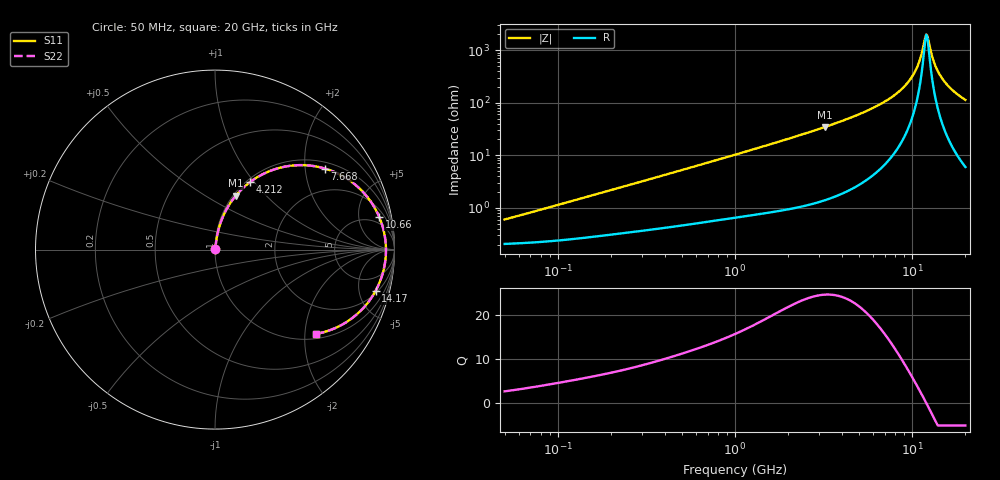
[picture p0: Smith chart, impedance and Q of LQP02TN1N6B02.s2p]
!Murata Part Number: LQP02TN1N6B02
!These Parameters are Measured in Series Mode Connection
!  o--[Z]--o
!Port1  Port2
!  o-------o
!Freq. Start=50[MHz] Stop=20[GHz], 401[Steps]
# Hz S RI R 50
!Freq.(Hz) S11(Real) S11(Imag) S21(Real) S21(Imag) S12(Real) S12(Imag) S22(Real) S22(Imag)
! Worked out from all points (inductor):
!   401 points, 50 MHz to 20 GHz, reference 50 ohm
!   read as one part in series: L = 1.79 nH near 56.37 MHz
!   highest Q = 24.7 at 3.217 GHz (marker M1), where L = 1.71 nH
!   self-resonance near 12.07 GHz
!   S11 on the Smith chart (normalised r, x): 50 MHz: 1.00, +0.01; 4.212 GHz: 1.04, +0.95; 7.668 GHz: 1.19, +2.55; 10.66 GHz: 3.27, +9.13; 14.17 GHz: 2.29, -7.18; 20 GHz: 1.12, -2.27
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5e7  0.00209 0.00563  0.9979 -0.00563  0.9979 -0.00563  0.00209 0.00563
1.364002e8  0.00288 0.0149  0.9971 -0.0149  0.9971 -0.0149  0.00288 0.0149
3.721004e8  0.00553 0.0388  0.9945 -0.0388  0.9945 -0.0388  0.00553 0.0388
1e9  0.0166 0.1  0.9834 -0.1  0.9834 -0.1  0.0166 0.1
2.728004e9  0.0853 0.2594  0.9147 -0.2594  0.9147 -0.2594  0.0853 0.2594
3.216634e9  0.1162 0.3008  0.8838 -0.3008  0.8838 -0.3008  0.1162 0.3008
4.212059e9  0.1957 0.3764  0.8043 -0.3764  0.8043 -0.3764  0.1957 0.3764
5.683258e9  0.3524 0.4535  0.6476 -0.4535  0.6476 -0.4535  0.3524 0.4535
7.442007e9  0.5816 0.4596  0.4184 -0.4596  0.4184 -0.4596  0.5816 0.4596
7.668323e9  0.6119 0.4518  0.3881 -0.4518  0.3881 -0.4518  0.6119 0.4518
9.316812e9  0.8108 0.3351  0.1892 -0.3351  0.1892 -0.3351  0.8108 0.3351
1.004137e10  0.8756 0.2559  0.1244 -0.2559  0.1244 -0.2559  0.8756 0.2559
1.066139e10  0.9159 0.1798  0.0841 -0.1798  0.0841 -0.1798  0.9159 0.1798
1.115139e10  0.9371 0.1169  0.0629 -0.1169  0.0629 -0.1169  0.9371 0.1169
1.183995e10  0.9515 0.0282  0.0485 -0.0282  0.0485 -0.0282  0.9515 0.0282
1.201863e10  0.9525 0.00558  0.0475 -0.00558  0.0475 -0.00558  0.9525 0.00558
1.238412e10  0.9511 -0.0397  0.0489 0.0397  0.0489 0.0397  0.9511 -0.0397
1.314879e10  0.9357 -0.1283  0.0643 0.1283  0.0643 0.1283  0.9357 -0.1283
1.417136e10  0.8947 -0.2302  0.1053 0.2302  0.1053 0.2302  0.8947 -0.2302
1.527346e10  0.8345 -0.3162  0.1655 0.3162  0.1655 0.3162  0.8345 -0.3162
1.646126e10  0.7621 -0.3832  0.2379 0.3832  0.2379 0.3832  0.7621 -0.3832
2e10  0.5601 -0.4707  0.4399 0.4707  0.4399 0.4707  0.5601 -0.4707
